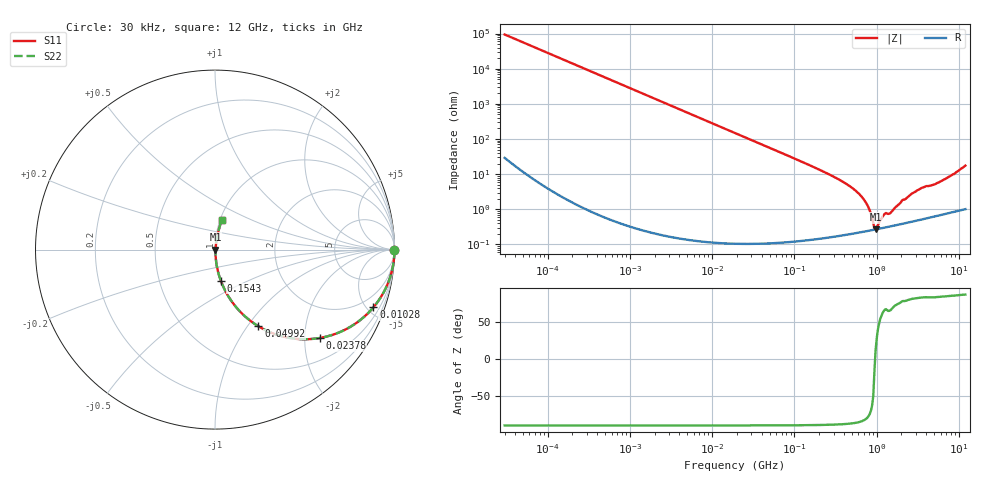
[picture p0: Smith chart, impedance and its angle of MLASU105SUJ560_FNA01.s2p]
! MLASU105SUJ560_FNA01  S-PARAMETER MODEL  ( General Type )
! Model Generated by TAIYO YUDEN Corporation (http://www.ty-top.com)
! Version 4.0
! TAIYO YUDEN Control No. 120810
! Copyright(c) 2003 TAIYO YUDEN CO.,LTD. All Rights Reserved.
! Product Description (link to TY-COMPAS)
! https://ds.yuden.co.jp/TYCOMPAS/or/detail?pn=MLASU105SUJ560JFNA01&u=M
! Products Name : Multilayer Ceramic Capacitors
! Characteristics :
!  Capacitance : 56 pF , Rated Voltage : 50V , TCC : UJ / U2J
!  Case Size : 1.0 x 0.5 / 0.039 x 0.02 [mm/inch] , Thickness : 0.5 / 0.02 [mm/inch]
!  (Conditions: Temperature = 25 degC , DC Bias Current/Voltage = 0A / 0V)
! External Node Assignments :
!  1  o---| |---o  2
! GND o---------o GND
! Frequency Range : 0.03MHz  -  12000MHz  [ 401 STEP ]
# MHz S RI R 50
! Freq[MHz].  S11 Real  S11 Imag  S21 Real  S21 Imag  S12 Real  S12 Imag  S22 Real  S22 Imag
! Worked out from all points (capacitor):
!   401 points, 30 kHz to 12 GHz, reference 50 ohm
!   read as one part in series: C = 56.3 pF near 32 kHz
!   lowest |Z| = 272 mohm at 970 MHz (marker M1)
!   series resonance near 958.9 MHz, so ESL is about 490 pH
!   S11 on the Smith chart (normalised r, x): 30 kHz: open; 10.28 MHz: 1.00, -5.49; 23.78 MHz: 1.00, -2.37; 49.92 MHz: 1.00, -1.13; 154.3 MHz: 1.00, -0.36; 12 GHz: 1.02, +0.35
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0.03  1 -0.00106  1.46e-06 0.00106  1.46e-06 0.00106  1 -0.00106
0.260295  0.9999 -0.00921  8.59e-05 0.00921  8.59e-05 0.00921  0.9999 -0.00921
2.258455  0.9936 -0.0794  0.00636 0.0794  0.00636 0.0794  0.9936 -0.0794
10.28143  0.8829 -0.3214  0.1171 0.3214  0.1171 0.3214  0.8829 -0.3214
18.97367  0.6888 -0.4626  0.3112 0.4626  0.3112 0.4626  0.6888 -0.4626
23.77866  0.5849 -0.4923  0.4151 0.4923  0.4151 0.4923  0.5849 -0.4923
49.92358  0.2419 -0.4273  0.7581 0.4273  0.7581 0.4273  0.2419 -0.4273
83.63502  0.1018 -0.3007  0.8982 0.3007  0.8982 0.3007  0.1018 -0.3007
154.3427  0.032 -0.1723  0.968 0.1723  0.968 0.1723  0.032 -0.1723
164.6252  0.0282 -0.1616  0.9718 0.1616  0.9718 0.1616  0.0282 -0.1616
368.6592  0.006 -0.0648  0.994 0.0648  0.994 0.0648  0.006 -0.0648
598.0015  0.00298 -0.0287  0.997 0.0287  0.997 0.0287  0.00298 -0.0287
774.0045  0.00257 -0.0127  0.9974 0.0127  0.9974 0.0127  0.00257 -0.0127
909.4299  0.0026 -0.00316  0.9974 0.00316  0.9974 0.00316  0.0026 -0.00316
970.0175  0.00267 0.000489  0.9973 -0.000489  0.9973 -0.000489  0.00267 0.000489
1001.808  0.00271 0.00138  0.9973 -0.00138  0.9973 -0.00138  0.00271 0.00138
1215.67  0.00301 0.00612  0.997 -0.00612  0.997 -0.00612  0.00301 0.00612
1428.372  0.00326 0.00677  0.9967 -0.00677  0.9967 -0.00677  0.00326 0.00677
2036.564  0.00413 0.0173  0.9959 -0.0173  0.9959 -0.0173  0.00413 0.0173
2903.719  0.00553 0.0303  0.9945 -0.0303  0.9945 -0.0303  0.00553 0.0303
5534.236  0.00961 0.0553  0.9904 -0.0553  0.9904 -0.0553  0.00961 0.0553
12000  0.0388 0.1662  0.9612 -0.1662  0.9612 -0.1662  0.0388 0.1662
